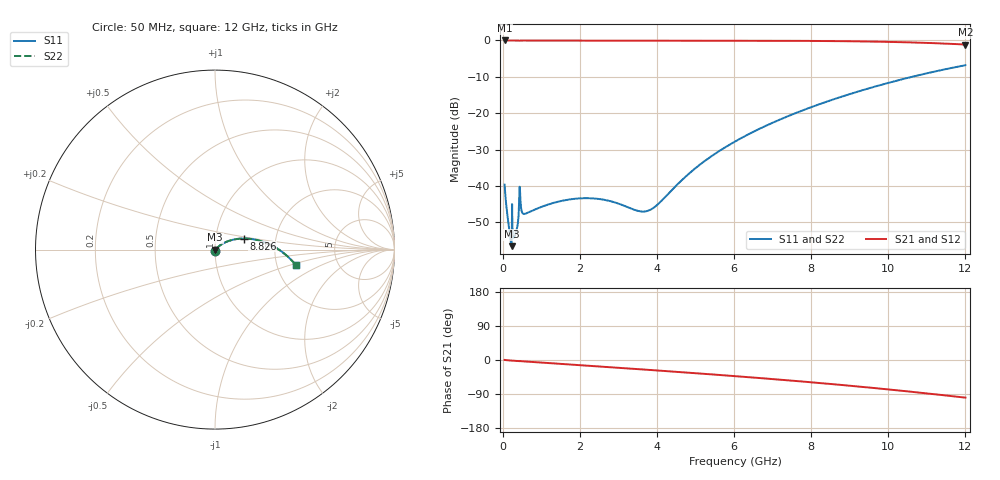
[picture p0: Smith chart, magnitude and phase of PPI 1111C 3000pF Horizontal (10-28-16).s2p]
# MHz S MA R 50
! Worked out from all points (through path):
!   1601 points, 50 MHz to 12 GHz, reference 50 ohm
!   highest |S21| = 0.00 dB at 50 MHz (marker M1); lowest = -1.1 dB at 12 GHz (marker M2)
!   group delay of S21, straight-line fit = 22.5 ps
!   lowest |S11| = -56.6 dB at 229.2 MHz (marker M3), VSWR 1.00, Z = 50.1 - j0.0678 ohm
!   |S11| at or under -10 dB: start of sweep to 10.62 GHz
!   |S22| runs from -56.6 to -6.8 dB; largest |S21 - S12| = 0
!   S11 on the Smith chart (normalised r, x): 50 MHz: 1.00, -0.02; 8.826 GHz: 1.37, +0.17; 12 GHz: 2.55, -0.54
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50  0.01041 -87.7  0.9996 0.2  0.9996 0.2  0.01041 -87.7
169.5  0.002551 -75.2  0.9993 -1.0  0.9993 -1.0  0.002551 -75.2
229.25  0.001485 -27.1  0.9986 -1.6  0.9986 -1.6  0.001485 -27.1
333.8125  0.00222 -18.1  0.9978 -2.3  0.9978 -2.3  0.00222 -18.1
363.6875  0.002535 -10.0  0.9975 -2.5  0.9975 -2.5  0.002535 -10.0
408.5  0.003694 7.6  0.9963 -2.9  0.9963 -2.9  0.003694 7.6
475.7188  0.00505 -53.5  0.9967 -3.1  0.9967 -3.1  0.00505 -53.5
528  0.004161 -47.5  0.997 -3.5  0.997 -3.5  0.004161 -47.5
580.2812  0.004145 -46.2  0.9969 -3.9  0.9969 -3.9  0.004145 -46.2
1357.031  0.00592 -62.7  0.9964 -9.2  0.9964 -9.2  0.00592 -62.7
2044.156  0.006759 -69.8  0.9961 -13.9  0.9961 -13.9  0.006759 -69.8
2708.875  0.006324 -68.7  0.9958 -18.5  0.9958 -18.5  0.006324 -68.7
3605.125  0.004446 -31.4  0.9954 -24.8  0.9954 -24.8  0.004446 -31.4
3814.25  0.004658 -11.6  0.9953 -26.2  0.9953 -26.2  0.004658 -11.6
4038.312  0.005674 7.9  0.9952 -27.8  0.9952 -27.8  0.005674 7.9
5001.781  0.01757 38.4  0.9945 -34.8  0.9945 -34.8  0.01757 38.4
6025  0.04075 39.5  0.9932 -42.6  0.9932 -42.6  0.04075 39.5
6943.656  0.07162 35.1  0.9908 -49.9  0.9908 -49.9  0.07162 35.1
8019.156  0.1219 27.7  0.9851 -58.9  0.9851 -58.9  0.1219 27.7
8825.781  0.171 21.2  0.9771 -66.2  0.9771 -66.2  0.171 21.2
10013.31  0.2619 10.3  0.9558 -77.8  0.9558 -77.8  0.2619 10.3
12000  0.4568 -10.7  0.8782 -99.3  0.8782 -99.3  0.4568 -10.7
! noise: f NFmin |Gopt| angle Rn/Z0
50  0.0004141  0.8788  0.355  0.0007389
1372  0.006732  0.8047  9.582  0.007114
2701  0.01007  0.7546  18.72  0.008073
4031  0.01297  0.728  27.58  0.008961
5360  0.01572  0.715  36.05  0.009875
6682  0.01844  0.7114  44.01  0.01087
8012  0.02126  0.715  51.5  0.01203
9341  0.02426  0.724  58.47  0.01339
1.067e+04  0.02753  0.7372  64.93  0.01505
1.2e+04  0.03116  0.7536  70.91  0.01711
